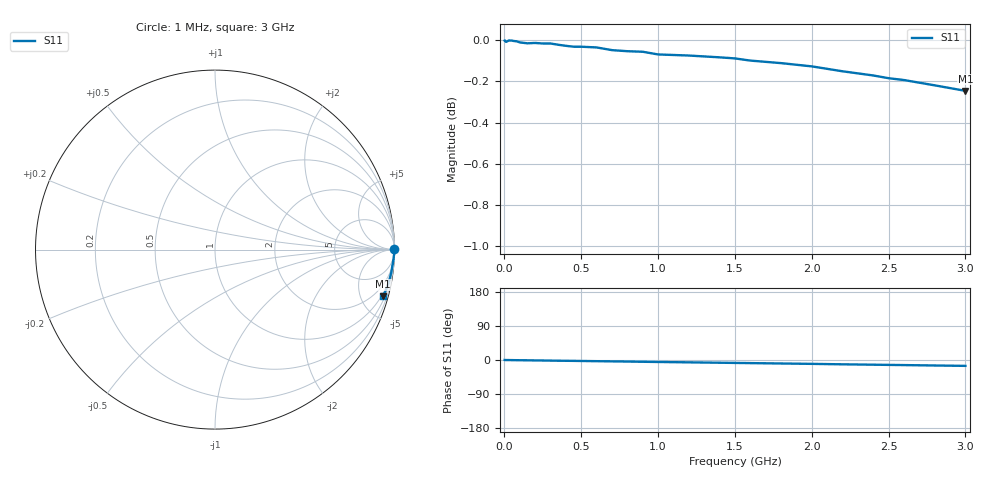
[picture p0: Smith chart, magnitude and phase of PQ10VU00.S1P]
! SIEMENS Small Signal Semiconductors
! BAR64-04
! Si PIN Diode in SOT23 (2 diodes in series, pin 3 open)
! VR = 10 V
! S-Parameters:  July  1992
# GHz  S  MA  R  50
!  f  S11
! GHz  MAG  ANG
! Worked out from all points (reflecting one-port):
!   33 points, 1 MHz to 3 GHz, reference 50 ohm
!   lowest |S11| = -0.2 dB at 3 GHz (marker M1), VSWR 70.68, Z = 38.5 - j363 ohm
!   phase of S11 starts at 0 deg and turns -16 deg over the sweep
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0.001  0.9998 0.1
0.003  0.9999 0.0
0.01  0.9991 -0.1
0.03  0.9999 -0.2
0.05  0.9998 -0.3
0.06  0.9996 -0.4
0.1  0.9988 -0.6
0.15  0.9983 -0.8
0.2  0.9985 -1.1
0.25  0.9982 -1.3
0.35  0.9975 -1.9
0.4  0.9969 -2.1
0.45  0.9964 -2.3
0.5  0.9964 -2.6
0.6  0.996 -3.1
0.7  0.9945 -3.6
0.8  0.9939 -4.1
0.9  0.9936 -4.7
1  0.9921 -5.2
1.2  0.9915 -6.2
1.5  0.9899 -7.7
1.6  0.9887 -8.2
2  0.9855 -10.2
2.2  0.9828 -11.4
2.4  0.9805 -12.4
2.6  0.978 -13.4
2.8  0.9751 -14.5
3  0.9721 -15.5
